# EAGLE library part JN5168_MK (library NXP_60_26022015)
IEEE802.15.4 Wireless Microcontroller The JN516x series is a range of ultra low power, high performance wireless microcontrollers suitable for JenNet-IP, ZigBee PRO, Remote Control, JenNet, and Active RFID applications. They feature an enhanced 32-bit RISC processor with embedded Flash and EEPROM memory, offering high coding efficiency through variable width instructions, a multi-stage instruction pipeline and low power operation with programmable clock speeds. They also include a 2.4GHz IEEE802.15.4 compliant transceiver and a comprehensive mix of analogue and digital peripherals. Three memory configurations are available to suit different applications. The best in class operating current is below 15mA, and, with a 0.6uA sleep timer mode, gives excellent battery life allowing operation direct from a coin cell. The peripherals support a wide range of applications. They include a 2-wire I2C, and SPI ports which can operate as either master or slave, a four channel ADC with battery and a temperature sensor. It can support a large switch matrix of up to 100 elements, or alternatively a 40 key capacitive touch pad. AAL Eindhoven MK
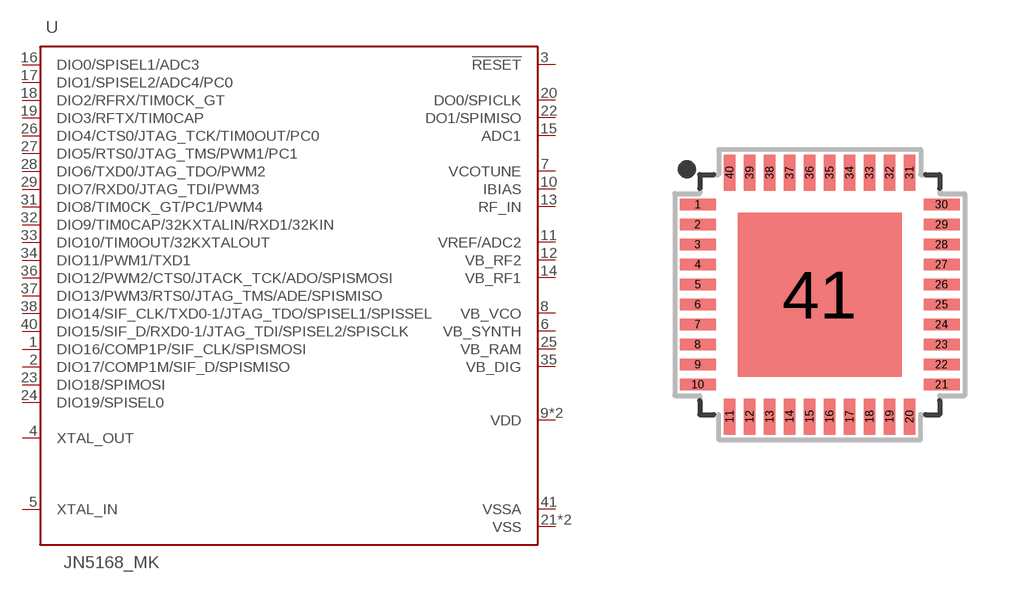
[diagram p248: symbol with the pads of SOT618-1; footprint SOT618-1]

Designator prefix U

## JN5168_MK (EEPROM: 4kB; FLASH: 256kB; RAM: 32kB)  [SOT618-1]
1  DIO16/COMP1P/SIF_CLK/SPISMOSI
2  DIO17/COMP1M/SIF_D/SPISMISO
3  !RESET!  in
4  XTAL_OUT  out
5  XTAL_IN  in
6  VB_SYNTH  pwr
7  VCOTUNE  pas
8  VB_VCO  pwr
9  VDD
10  IBIAS  pas
11  VREF/ADC2  pas
12  VB_RF2  pwr
13  RF_IN  pas
14  VB_RF1  pwr
15  ADC1  pas
16  DIO0/SPISEL1/ADC3
17  DIO1/SPISEL2/ADC4/PC0
18  DIO2/RFRX/TIM0CK_GT
19  DIO3/RFTX/TIM0CAP
20  DO0/SPICLK  out
21  VSS  pwr
22  DO1/SPIMISO  in
23  DIO18/SPIMOSI
24  DIO19/SPISEL0
25  VB_RAM  pwr
26  DIO4/CTS0/JTAG_TCK/TIM0OUT/PC0
27  DIO5/RTS0/JTAG_TMS/PWM1/PC1
28  DIO6/TXD0/JTAG_TDO/PWM2
29  DIO7/RXD0/JTAG_TDI/PWM3
30  VDD
31  DIO8/TIM0CK_GT/PC1/PWM4
32  DIO9/TIM0CAP/32KXTALIN/RXD1/32KIN
33  DIO10/TIM0OUT/32KXTALOUT
34  DIO11/PWM1/TXD1
35  VB_DIG  pwr
36  DIO12/PWM2/CTS0/JTACK_TCK/ADO/SPISMOSI
37  DIO13/PWM3/RTS0/JTAG_TMS/ADE/SPISMISO
38  DIO14/SIF_CLK/TXD0-1/JTAG_TDO/SPISEL1/SPISSEL
39  VSS  pwr
40  DIO15/SIF_D/RXD0-1/JTAG_TDI/SPISEL2/SPISCLK
41  VSSA  pwr

## Footprint SOT618-1 (pad centres in mm)
SOT618-1 HVQFN40: plastic thermal enhanced very thin quad flat package; no leads; 40 terminals; body 6 x 6 x 0.85 mm JEDEC: MO-220 IEC: --
smd 0.9 x 0.29: 1 -3.05,2.25; 2 -3.05,1.75; 3 -3.05,1.25; 4 -3.05,0.75; 5 -3.05,0.25; 6 -3.05,-0.25; 7 -3.05,-0.75; 8 -3.05,-1.25; 9 -3.05,-1.75; 10 -3.05,-2.25; 21 3.05,-2.25; 22 3.05,-1.75; 23 3.05,-1.25; 24 3.05,-0.75; 25 3.05,-0.25; 26 3.05,0.25; 27 3.05,0.75; 28 3.05,1.25; 29 3.05,1.75; 30 3.05,2.25
smd 0.29 x 0.9: 11 -2.25,-3.05; 12 -1.75,-3.05; 13 -1.25,-3.05; 14 -0.75,-3.05; 15 -0.25,-3.05; 16 0.25,-3.05; 17 0.75,-3.05; 18 1.25,-3.05; 19 1.75,-3.05; 20 2.25,-3.05; 31 2.25,3.05; 32 1.75,3.05; 33 1.25,3.05; 34 0.75,3.05; 35 0.25,3.05; 36 -0.25,3.05; 37 -0.75,3.05; 38 -1.25,3.05; 39 -1.75,3.05; 40 -2.25,3.05
smd 4.1 x 4.1: 41 0,0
